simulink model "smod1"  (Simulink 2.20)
settings: Solver=ode45  StartTime=0.0  StopTime=6.0  RelTol=1e-3  AbsTol=1e-6
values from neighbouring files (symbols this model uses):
  h = 0.1    [demo_04.m]    (also in demo_smod1.m; demo_stvmod.m = 1; demo_reces01.m = 1; demo_reces03.m = 1)
  K = 2    [demo_smod1.m]    (also in demo_astrejc.m = 1; demo_strejc.m = 1; rarxcup.m = P*phi(i)/(1+phi(i)'*P*phi(i)); rarxm_ml.m = w/(ff+phi(i)'*w))
  T1 = 1    [demo_smod1.m]    (also in demo_astrejc.m = 10; demo_strejc.m = 10)
  T2 = 0.5    [demo_smod1.m]    (also in demo_astrejc.m = 5; demo_strejc.m = 5)

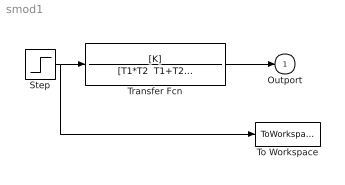
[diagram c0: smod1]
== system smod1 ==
  Step : Step  Time=0  Before=0  After=1
  To Workspace : ToWorkspace  VariableName=u  SampleTime=h
  Transfer Fcn : TransferFcn  Numerator=[K]  Denominator="[T1*T2  T1+T2  1]"
  Outport : Outport  Port=1  InitialOutput=0
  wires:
  Transfer Fcn/1 -> Outport/1
  Step/1 -> Transfer Fcn/1, To Workspace/1
